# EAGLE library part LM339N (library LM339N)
Quad Differential Comparator Source: Datasheet
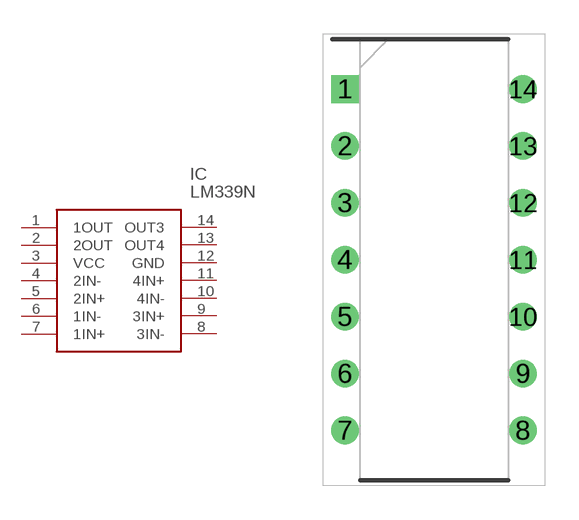
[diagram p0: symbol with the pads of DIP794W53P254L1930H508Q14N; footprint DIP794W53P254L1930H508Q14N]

Designator prefix IC

## LM339N (Arrow_Part_Number: LM339N; Arrow_Price-Stock: https://www.arrow.com/en/products/lm339n/texas-instruments?region=nac; Description: Quad Differential Comparator; Height: 5.08mm; Manufacturer_Name: Texas Instruments; Manufacturer_Part_Number: LM339N; Mouser_Part_Number: 595-LM339N; Mouser_Price-Stock: https://www.mouser.co.uk/ProductDetail/Texas-Instruments/LM339N?qs=rshUhwi3fbY%252BaR%252BOl3edNw%3D%3D)  [DIP794W53P254L1930H508Q14N]
1  1OUT
2  2OUT
3  VCC
4  2IN-
5  2IN+
6  1IN-
7  1IN+
8  3IN-
9  3IN+
10  4IN-
11  4IN+
12  GND
13  OUT4
14  OUT3

## Footprint DIP794W53P254L1930H508Q14N (pad centres in mm)
LM339N
drill 0.73 pad 1.13 square: 1 -3.97,7.62
drill 0.73 pad 1.13: 2 -3.97,5.08; 3 -3.97,2.54; 4 -3.97,0; 5 -3.97,-2.54; 6 -3.97,-5.08; 7 -3.97,-7.62; 8 3.97,-7.62; 9 3.97,-5.08; 10 3.97,-2.54; 11 3.97,0; 12 3.97,2.54; 13 3.97,5.08; 14 3.97,7.62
